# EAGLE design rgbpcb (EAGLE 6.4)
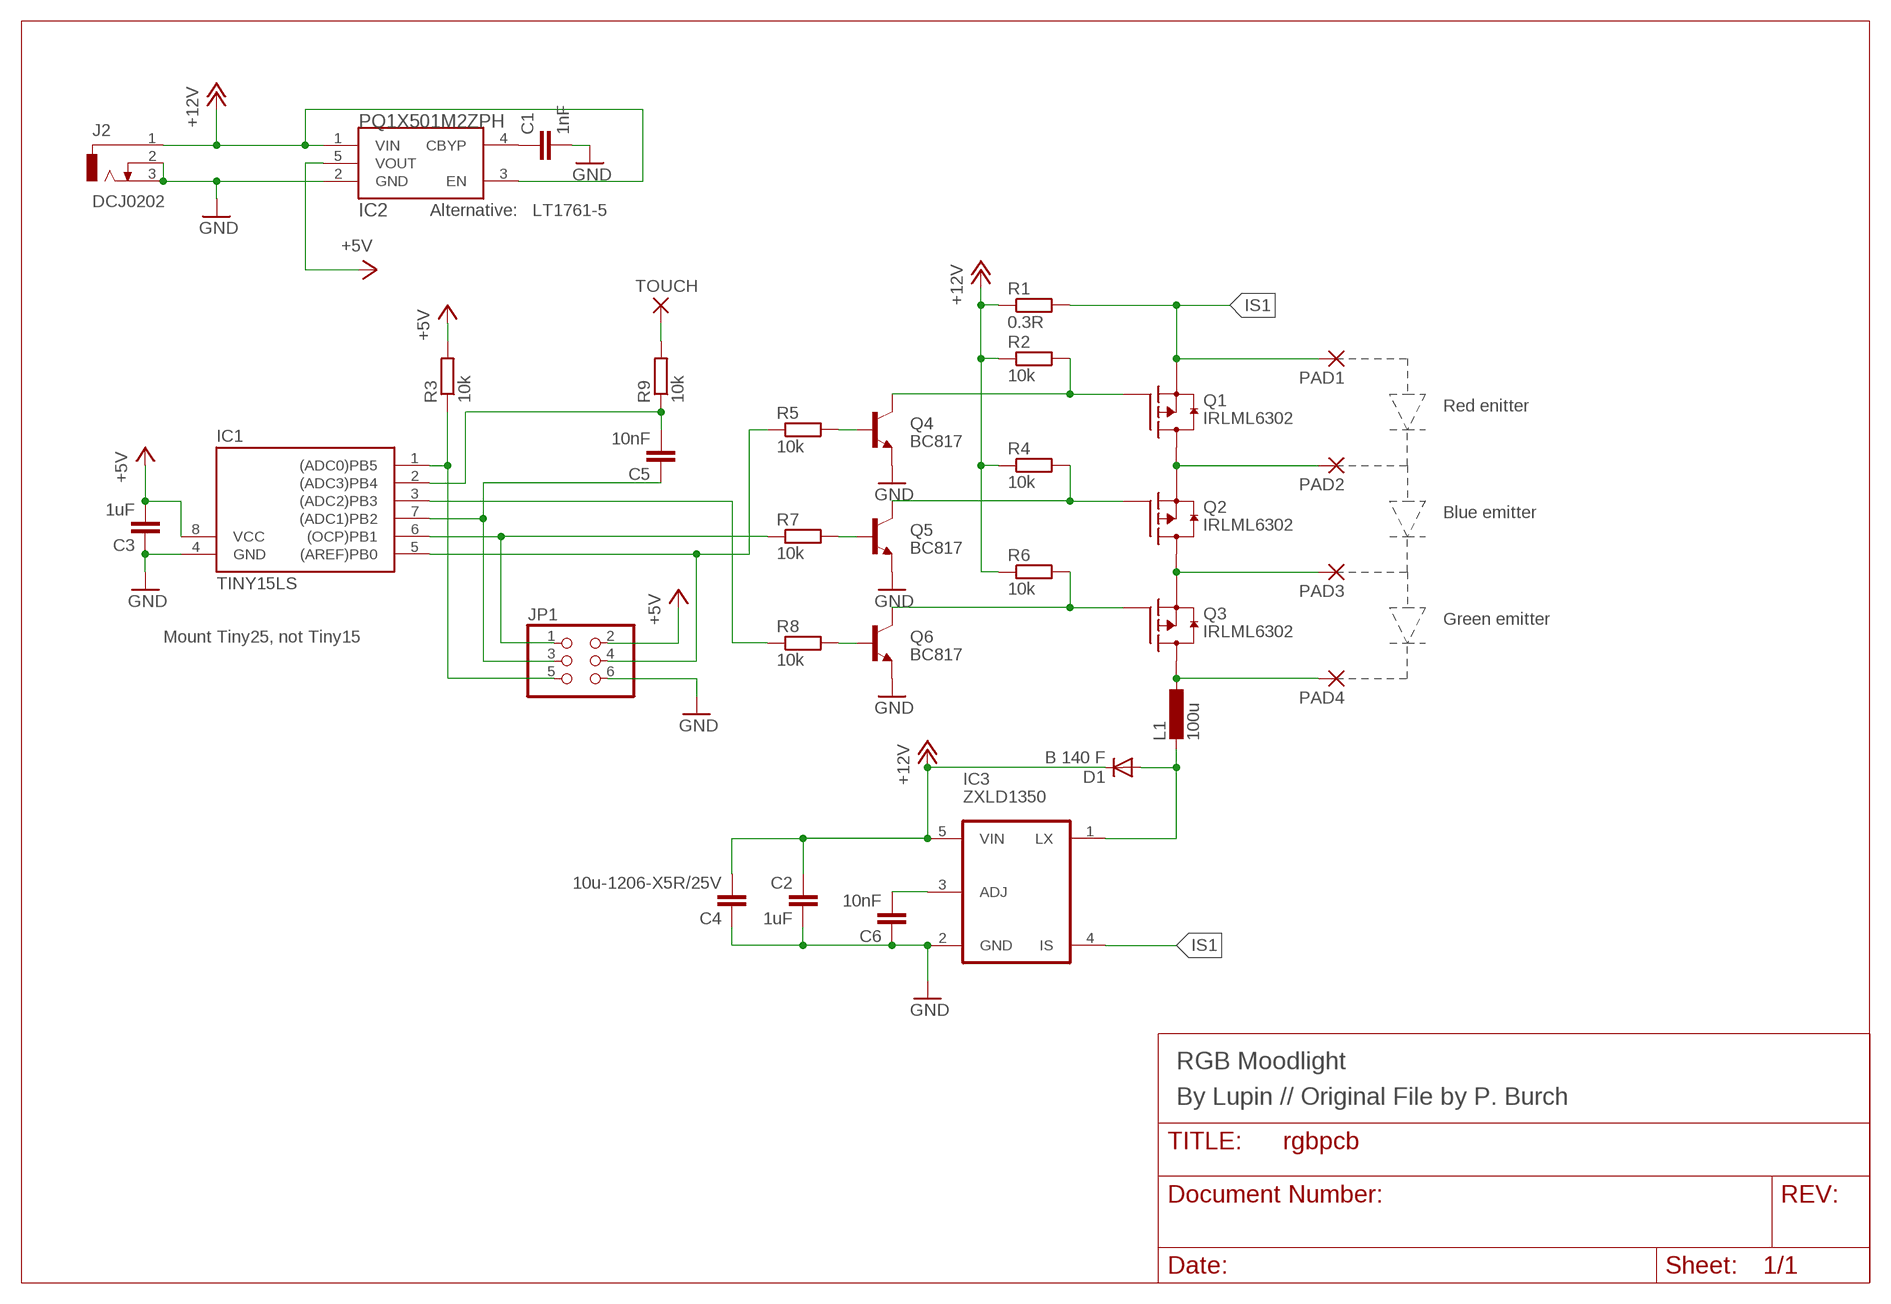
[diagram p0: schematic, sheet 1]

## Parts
C1  1nF  C-EUC0603  [C0603]
C2  1uF  C-EUC0603  [C0603]
C3  1uF  C-EUC0603  [C0603]
C4  10u-1206-X5R/25V  C-EUC1206  [C1206]
C5  10nF  C-EUC0603  [C0603]
C6  10nF  C-EUC0603  [C0603]
D1  B 140 F  DIODE-DO-214AC  [DO-214AC]
IC1  TINY15LS  [SOIC8]
IC2  PQ1X501M2ZPH  IRU1205-33  [SOT23-5]
IC3  ZXLD1350  [SOT23-5]
J2  DCJ0202  [DCJ0202]
JP1  PINHD-2X3_2.54-SMD  [2X03SMD]
L1  100u  L-EUPIS2816  [PIS2816]
PAD1  SMD2  [SMD1,27-2,54]
PAD2  SMD2  [SMD1,27-2,54]
PAD3  SMD2  [SMD1,27-2,54]
PAD4  SMD2  [SMD1,27-2,54]
Q1  IRLML6302  [SOT23]
Q2  IRLML6302  [SOT23]
Q3  IRLML6302  [SOT23]
Q4  BC817  BC817-40SMD  [SOT23-BEC]
Q5  BC817  BC817-40SMD  [SOT23-BEC]
Q6  BC817  BC817-40SMD  [SOT23-BEC]
R1  0.3R  R-EU_R1206  [R1206]
R2  10k  R-EU_R0603  [R0603]
R3  10k  R-EU_R0603  [R0603]
R4  10k  R-EU_R0603  [R0603]
R5  10k  R-EU_R1206  [R1206]
R6  10k  R-EU_R0603  [R0603]
R7  10k  R-EU_R1206  [R1206]
R8  10k  R-EU_R1206  [R1206]
R9  10k  R-EU_R0603  [R0603]
TOUCH  SMD2  [SMD1,27-2,54]

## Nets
+5V: C3.2 IC1.8(VCC) IC2.5(VOUT) JP1.2 R3.2
+12V: C2.1 C4.2 D1.C IC2.1(VIN) IC2.3(EN) IC3.5(VIN) J2.1 R1.1 R2.1 R4.1 R6.1
GND: C1.2 C2.2 C3.1 C4.1 C6.1 IC1.4(GND) IC2.2(GND) IC3.2(GND) J2.2 J2.3 JP1.6 Q4.E Q5.E Q6.E
IS1: IC3.4(IS) PAD1.1(P) Q1.2(S) R1.2
N$1: Q2.1(G) Q5.C R4.2
N$2: Q3.1(G) Q6.C R6.2
N$3: D1.A IC3.1(LX) L1.2
N$4: C1.1 IC2.4(CBYP)
N$5: IC1.6((OCP)PB1) JP1.1 R7.1
N$6: Q4.B R5.2
N$7: Q1.1(G) Q4.C R2.2
N$8: IC1.1((ADC0)PB5) JP1.5 R3.1
N$9: Q5.B R7.2
N$10: C5.1 IC1.7((ADC1)PB2) JP1.3
N$11: Q6.B R8.2
N$12: R9.2 TOUCH.1(P)
N$13: C5.2 IC1.2((ADC3)PB4) R9.1
N$14: C6.2 IC3.3(ADJ)
OUT1: PAD2.1(P) Q1.3(D) Q2.2(S)
OUT2: PAD3.1(P) Q2.3(D) Q3.2(S)
OUT3: L1.1 PAD4.1(P) Q3.3(D)
PWM1: IC1.5((AREF)PB0) JP1.4 R5.1
PWM3: IC1.3((ADC2)PB3) R8.1

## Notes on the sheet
- Alternative:   LT1761-5
- Red enitter
- Blue emitter
- Green emitter
- Mount Tiny25, not Tiny15
- RGB Moodlight
- By Lupin // Original File by P. Burch

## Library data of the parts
C1-C6 = rcl:C-EU: CAPACITOR, European symbol
D1 = diode:DIODE-: DIODE
IC1 = atmel:TINY15L: MICROCONTROLLER 2.7 V 1 Kbytes FLASH 64 bytes EEPROM 4-channel 10 bit ADC
IC2 = iru:IRU1205-33
IC3 = zetex:ZXLD1350: 350mA LED driver with internal switch Features: Supply voltage up to 30V High efficiency up to 95% Up to 1MHz switching frequency
J2 = con-jack:DCJ0202: DC POWER JACK Source: DCJ0202.pdf
JP1 = pinheadsmd:PINHD-2X3: PIN HEADER
L1 = rcl:L-EU: INDUCTOR, European symbol
PAD1-PAD4 TOUCH = wirepad:SMD2: SMD PAD
Q1-Q3 = transistor-fet:IRLML6302: P-Channel Enhancement MOSFET (HEXFET) RDSOn = 0.6R VDS = -20V IDS = 780mA
Q4-Q6 = transistor-npn:BC817*: NPN Transistor
R1-R9 = rcl:R-EU_: RESISTOR, European symbol

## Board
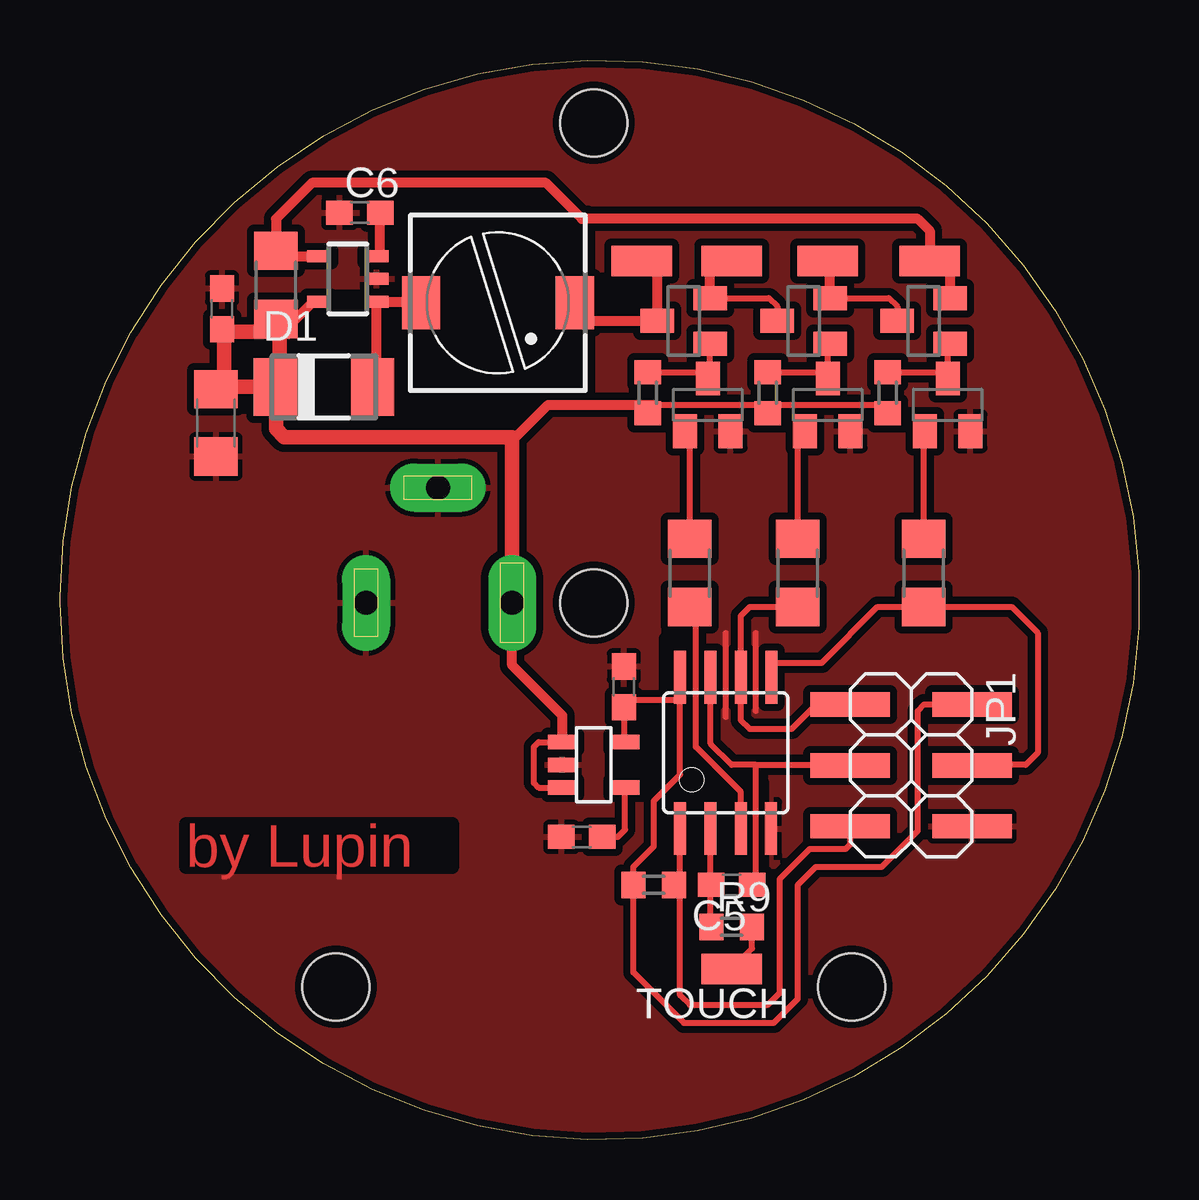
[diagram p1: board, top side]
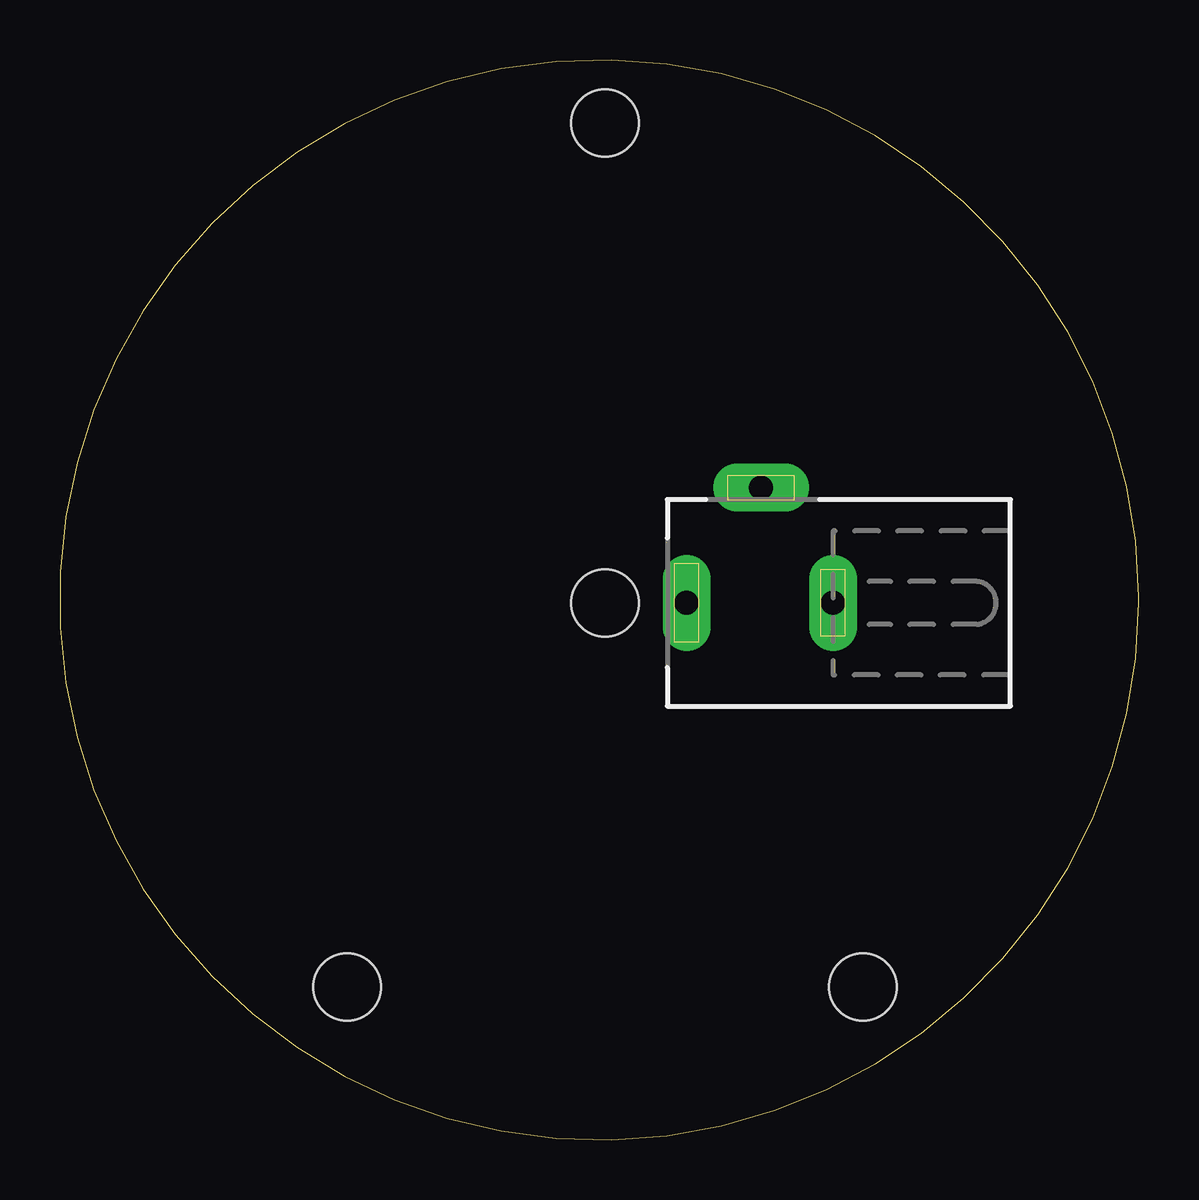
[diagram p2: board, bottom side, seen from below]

Size 44.97 x 44.99 mm. Coordinates in mm from the lower left corner, seen from the top.
Outline: 0,22.62 arc-359 0,22.37 0,22.62
Copper layers (1*16): Top 0.035mm / dielectric 1.5mm / Bottom 0.035mm
Design rules "PCB-POOL *": minimum track width 8mil, minimum drill 12mil, track to track 8mil, track to pad 8mil, pad to pad 8mil, via to via 8mil, smd to smd 0mil, copper to edge 0.1mm, drill to drill 8mil, minimum pad ring 8mil, minimum via ring 6mil, stop-mask expansion 3mil, vias tented up to drill 0mil, thermal gap 8mil
Holes 2.8 mm at 22.25,42.37 11.5,6.37 33,6.37 22.25,22.37
tRestrict: area 14.5,31.1 to 22,38.6; area 28.5,11.4 to 29.2,14.9; area 25.2,15.4 to 26.5,20.9; area 23,15.1 to 24,16.1; area 10.5,34.1 to 13.5,35.1

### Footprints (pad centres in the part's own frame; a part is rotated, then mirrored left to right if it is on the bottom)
C0603 = smd 1.1 x 1: 1 -0.85,0; 2 0.85,0
C1206 = smd 1.6 x 1.8: 1 -1.4,0; 2 1.4,0
DO-214AC = smd 1.8 x 2.4: A 2.025,0; C -2.025,0
SOIC8 = smd 0.5 x 2.2: 1 -1.905,-3.154; 2 -0.645,-3.154; 3 0.625,-3.154; 4 1.895,-3.154; 5 1.905,3.154; 6 0.635,3.154; 7 -0.635,3.154; 8 -1.905,3.154
SOT23-5 = smd 0.6 x 1.2: 1 -0.95,-1.306; 2 0,-1.306; 3 0.95,-1.306; 4 0.95,1.306; 5 -0.95,1.306
SOT23-5' = smd 0.5 x 1: 1 -0.95,-1.2; 2 0,-1.2; 3 0.95,-1.2; 4 0.95,1.2; 5 -0.95,1.2
DCJ0202 = drill 1 pad 2 long: 1 0,3.1; 2 4.8,0; 3 0,-3
2X03SMD = smd 1.016 x 3.302: 1 -1.27,-3.81; 2 -1.27,1.27; 3 1.27,-3.81; 4 1.27,1.27; 5 3.81,-3.81; 6 3.81,1.27
PIS2816 = smd 2.2 x 1.6: 1 0,3.2; 2 0,-3.2
SMD1,27-2,54 = smd 1.27 x 2.54: 1 0,0
SOT23 = smd 1 x 1.4: 1 -0.95,-1.1; 2 0.95,-1.1; 3 0,1.1
SOT23-BEC = smd 1 x 1.4: B -0.95,-1.1; C 0,1.1; E 0.95,-1.1
R1206 = smd 1.6 x 1.803: 1 -1.422,0; 2 1.422,0
R0603 = smd 1 x 1.1: 1 -0.85,0; 2 0.85,0

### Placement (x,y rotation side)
C1  21.75,12.62 180 top
C2  6.75,34.62 90 top
C3  23.5,18.87 270 top
C4  6.5,29.87 90 top
C5  28,10.62 180 top
C6  12.5,38.62 0 top
D1  11,31.37 0 top
IC1  27.75,16.12 0 top
IC2  22.25,15.62 270 top
IC3  ZXLD1350  [SOT23-5']  12,35.87 90 top
J2  15.75,22.37 90 bottom
JP1  36.75,16.87 270 top
L1  18.25,34.87 270 top
PAD1  36.25,36.62 90 top
PAD2  32,36.62 90 top
PAD3  28,36.62 90 top
PAD4  24.25,36.62 270 top
Q1  36,34.12 90 top
Q2  31,34.12 90 top
Q3  26,34.12 90 top
Q4  37,30.62 0 top
Q5  32,30.62 0 top
Q6  27,30.62 0 top
R1  9,35.62 90 top
R2  34.5,31.12 90 top
R3  24.75,10.62 180 top
R4  29.5,31.12 90 top
R5  36,23.62 90 top
R6  24.5,31.12 90 top
R7  30.75,23.62 90 top
R8  26.25,23.62 90 top
R9  28,8.87 0 top
TOUCH  28,7.12 90 top

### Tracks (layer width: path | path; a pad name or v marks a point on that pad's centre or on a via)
+5V
  Top 0.254: 23.75,18.32 25.89,18.32 IC1.8 25.84,15.21 24.75,14.12 24.75,12.22 23.9,11.37 R3.2 23.9,6.97 26,4.87 29.75,4.87 30.75,5.87 30.75,10.62 31.5,11.37 34.25,11.37 35.75,12.87 35.75,17.87 36.02,18.14 JP1.2 | C3.2 23.9,17.97 23.75,18.32 | IC2.5 23.44,16.56 23.5,16.62 C3.2 | 23.75,18.32 C3.2
+12V
  Top 0.254: 34.15,30.62 R2.1 34.4,30.62 29.25,30.62 | 29.25,30.62 24.75,30.62 R6.1 | 29.25,30.62 R4.1 | IC2.1 19.95,16.57 19.75,16.37 19.75,14.87 19.95,14.67 IC2.3
  Top 0.406: 18.85,29.12 20.35,30.62 24.75,30.62 | 9.5,33.67 R1.1 | IC2.1 20.94,17.68 18.85,19.77 J2.1 | IC3.5 10.54,34.92 9.15,33.52
  Top 0.61: 6.85,33.67 9.5,33.67 | J2.1 18.85,29.12 18.85,29.27 9.35,29.27 9,29.62 9,31.34 D1.C | D1.C 6.85,31.37 | 6.85,31.37 C4.2 | 6.85,31.37 6.85,33.67 | 6.85,33.67 C2.1 | 9.15,33.52 9.15,31.54 D1.C
GND
  Top 0.254: 27.75,17.62 27.75,21.12 | 29,17.87 29,21.12
  pour Top (isolate 0.305): 0,45.62 45.25,45.62 45.25,-0.13 0,-0.13
IS1
  Top 0.406: R1.2 9,37.62 | Q1.2 37.1,36.27 PAD1.1 36.25,37.87 35.75,38.37 21.75,38.37 20.25,39.87 10.5,39.87 9,38.37 R1.2 | IC3.4 9.72,36.82 R1.2
N$1
  Top 0.254: R4.2 31.5,31.97 Q5.C 32,32.82 Q2.1
N$2
  Top 0.254: R6.2 27,31.97 | 27,31.97 27.1,31.97 Q3.1 | 27,31.97 Q6.C
N$3
  Top 0.406: L1.2 15,34.92 IC3.1 13.2,31.44 D1.A
N$4
  Top 0.254: C1.1 23.25,12.62 23.56,12.93 IC2.4
N$5
  Top 0.254: JP1.1 32.42,18.12 31.5,18.12 30.5,17.12 28.75,17.12 28.39,17.48 IC1.6 28.39,21.83 28.75,22.2 R7.1
N$6
  Top 0.254: R5.2 36,29.22 Q4.B
N$7
  Top 0.254: R2.2 36.75,31.97 Q4.C 37,33.07 Q1.1
N$8
  Top 0.254: IC1.1 25.84,12.72 25.85,12.72 25.85,10.87 R3.1 25.85,10.37 25.85,6.02 26.25,5.62 29.5,5.62 30,6.12 30,10.87 31.25,12.12 32.75,12.12 32.94,12.31 JP1.5
N$9
  Top 0.254: R7.2 30.75,29.47 Q5.B
N$10
  Top 0.254: IC1.7 27.11,16.5 28,15.62 29,15.62 | 29,15.62 31.67,15.62 JP1.3 | C5.1 29,10.62 29,15.62
N$11
  Top 0.254: R8.2 26.25,29.47 Q6.B
N$12
  Top 0.254: R9.2 28.85,7.97 TOUCH.1
N$13
  Top 0.254: 27.11,10.62 C5.2 | 27.11,10.62 IC1.2 | 27.11,10.62 27.11,9.16 R9.1
N$14
  Top 0.406: IC3.3 13.35,36.82 C6.2
OUT1
  Top 0.254: Q2.2 34.55,35.07 34.9,34.72 Q1.3
  Top 0.406: Q2.2 32.1,36.27 PAD2.1
OUT2
  Top 0.254: Q3.2 29.55,35.07 29.9,34.72 Q2.3 | 27.1,36.52 PAD3.1
  Top 0.406: Q3.2 27.1,36.52
OUT3
  Top 0.254: 24.9,36.47 PAD4.1
  Top 0.406: 24.9,36.47 Q3.3 21.75,34.12 21.5,34.37 L1.1
PWM1
  Top 0.254: JP1.4 38.04,15.62 40.25,15.62 40.75,16.12 40.75,21.12 39.67,22.2 R5.1 34.08,22.2 31.75,19.87 29.75,19.87 29.66,19.77 IC1.5
PWM3
  Top 0.254: IC1.3 28.38,14.49 26.5,16.37 26.5,21.87 25.92,22.45 R8.1

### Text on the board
Top: by Lupin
